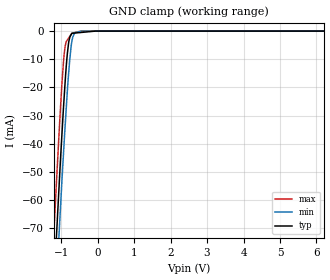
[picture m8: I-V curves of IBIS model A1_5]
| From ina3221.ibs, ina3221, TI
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[Model]   A1_5
Model_type   Input
Vinl = 1.5   |min, GND -0.5 V
Vinh = 3.5   |max. V+ 6 V
|   typ   min   max
|   (nom PVT)   (Fast PVT)   (slow PVT)
C_comp   5.599E-13   5.547E-13   5.971E-13
| Where   nom PVT is  Nominal Process, 3.3V, 25C
|   Fast PVT is Strong Process, 3.6V, -40C
|   Slow PVT is Weak Process, 3.0V, 85C
|C_comp - from L-C Tank method, L = 1nH, peak frequency
[Model Spec]
| variable   typ   min   max
Vinl   1.5   1.35   1.65
Vinh   3.5   3.15   3.85
|Vinl = 0.3 x V+, Vinh = 0.7 x V+
[Voltage Range]   5   4.5   5.5
|Ambient Temperature Range   27   85   -40
[Temperature Range]   30   88   -40
[Power Clamp Reference]   5   4.5   5.5
[GND Clamp Reference]   0   0   0
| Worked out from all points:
|   GND clamp passes 1 mA (typ) near -0.72 V on its own axis
[GND Clamp]
|   Voltage   I(typ)   I(min)   I(max)
-5V       -1.111A    -1.111A    -1.112A
-1.23V    -97.87mA   -113.9mA   -79.44mA
-1.131V   -73.49mA   -90.01mA   -54.25mA
-1.04V    -51.13mA   -68.06mA   -32.3mA
-980.8mV  -37.34mA   -53.79mA   -19.29mA
-920.4mV  -24.21mA   -40.24mA   -8.706mA
-862.7mV  -13.06mA   -28.08mA   -3.821mA
-797mV    -4.411mA   -15.56mA   -2.529mA
-707mV    -797.3uA   -3.787mA   -833.3uA
-624.4mV  -696.4uA   -567.2uA   -533.2uA
-434.8mV  -464.7uA   -3.534uA   -3.641uA
9.985V    0A         0A         0A
[POWER Clamp]
|   SCR cell for ESD function. Effects occurr above VDD x 2
|   Voltage   I(typ)   I(min)   I(max)
-5V       0A         0A         0A
0V        0A         0A         0A
10V       0A         0A         0A
